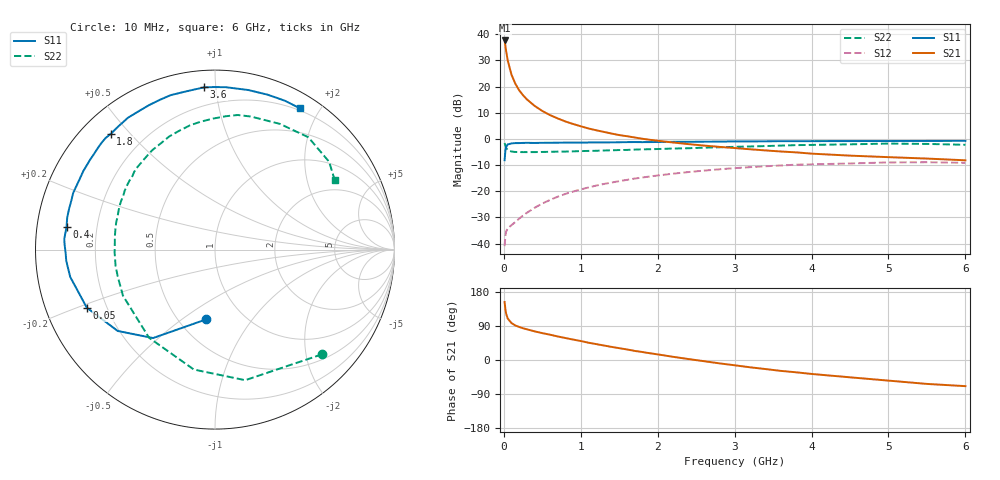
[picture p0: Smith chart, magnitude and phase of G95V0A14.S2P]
! SIEMENS Small Signal Semiconductors
! BFG235
! Si NPN RF Bipolar Junction Transistor in SOT223
! VCE = 5 V  IC = 140 mA
! Common Emitter S-Parameters:  July  1994
# GHz  S  MA  R  50
!  f  S11  S21  S12  S22
! GHz  MAG  ANG  MAG  ANG  MAG  ANG  MAG  ANG
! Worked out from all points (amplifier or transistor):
!   40 points, 10 MHz to 6 GHz, reference 50 ohm
!   highest |S21| = 37.6 dB at 10 MHz (marker M1)
!   |S21| within 3 dB of that: start of sweep to 24.67 MHz
!   unconditionally stable (mu >= 1): 472.9 MHz to 1.497 GHz
!   at 200 MHz: K = 0.81, MSG = 24.5 dB, |S12| = -30.5 dB
!   at 1.5 GHz: K = 1.00, MSG = 8.8 dB, |S12| = -16.1 dB
!   at 6 GHz: K = 0.89, MSG = 0.5 dB, |S12| = -9.2 dB
!   S11 on the Smith chart (normalised r, x): 10 MHz: 0.68, -0.62; 50 MHz: 0.13, -0.21; 400 MHz: 0.09, +0.07; 1.8 GHz: 0.08, +0.44; 3.6 GHz: 0.09, +0.93; 6 GHz: 0.17, +1.75
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0.01  0.3912 -97.0  76.28 153.0  0.0089 64.1  0.834 -44.4
0.02  0.6016 -125.0  60.32 134.2  0.0142 49.1  0.7468 -77.0
0.03  0.7066 -140.1  47.6 122.3  0.017 41.6  0.6785 -100.0
0.05  0.7841 -155.6  31.81 109.6  0.0195 34.5  0.6134 -126.8
0.1  0.8209 -169.3  16.83 97.3  0.0225 37.6  0.5735 -153.4
0.15  0.8311 -175.7  11.31 91.1  0.0258 43.1  0.5623 -164.5
0.2  0.8325 -178.9  8.47 87.1  0.03 48.2  0.5614 -170.7
0.25  0.8386 178.1  6.817 83.7  0.0343 51.4  0.559 -175.0
0.3  0.8418 175.9  5.699 81.0  0.0387 53.9  0.5595 -178.6
0.4  0.8367 171.4  4.28 75.6  0.0482 56.7  0.5594 176.2
0.5  0.8425 167.8  3.421 70.9  0.0582 58.2  0.563 172.0
0.7  0.8459 161.0  2.462 62.1  0.0786 57.7  0.571 164.6
0.9  0.8496 155.6  1.929 53.9  0.0984 54.9  0.5785 158.4
1.1  0.8543 149.2  1.584 45.6  0.1181 51.6  0.5895 152.3
1.4  0.8588 142.0  1.266 34.6  0.1463 45.8  0.6066 143.9
1.8  0.8678 132.1  1.008 21.1  0.183 37.2  0.6314 133.0
2.2  0.8803 123.4  0.854 8.4  0.2163 28.2  0.6547 122.4
3.2  0.895 102.0  0.634 -19.2  0.2885 5.0  0.7168 96.5
3.6  0.9059 93.8  0.575 -28.7  0.3107 -4.9  0.7454 85.4
4.5  0.9082 78.2  0.479 -45.7  0.3396 -24.6  0.7882 62.7
5.5  0.9163 64.9  0.421 -63.1  0.3583 -46.5  0.8023 37.6
6  0.9183 59.0  0.39 -69.0  0.3487 -54.8  0.7718 30.3
